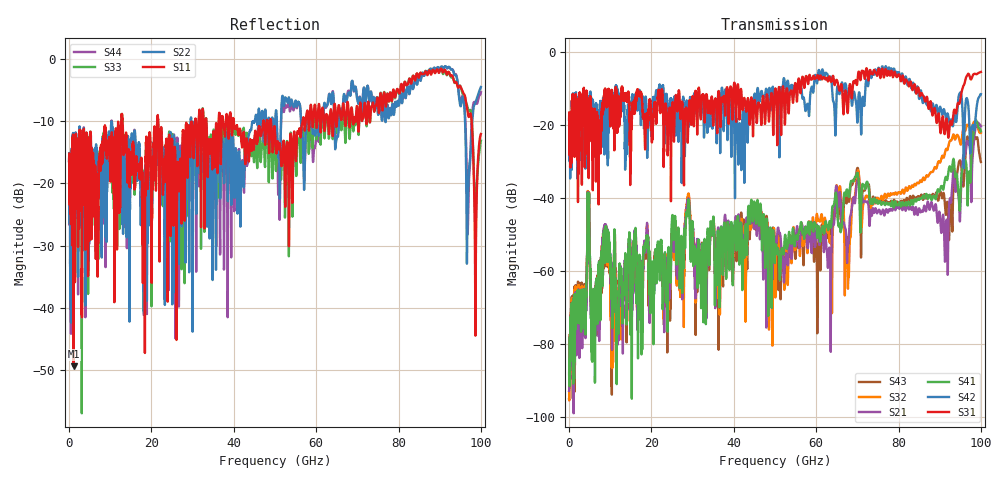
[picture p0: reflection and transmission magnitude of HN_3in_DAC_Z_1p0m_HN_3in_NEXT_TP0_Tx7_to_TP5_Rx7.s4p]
# GHz S RI R 45
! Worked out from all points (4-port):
!   4000 points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, 25 MHz to 100 GHz, reference 45 ohm
!   strongest paths, dB at 25 MHz, 25.02 GHz, 50.02 GHz, 75.03 GHz, 100 GHz:
!     S31: -18.6, -14.9, -10.3, -5.2, -5.5
!     S42: -18.6, -16.6, -12.4, -4.6, -11.5
!     S41: -88.3, -45.2, -55.9, -41.6, -21.7
!     S21: -92.8, -49.6, -53.3, -43.6, -20.4
!     S32: -95.1, -50.6, -58.0, -40.0, -22.2
!     S43: -95.0, -46.6, -57.9, -40.4, -30.1
!   lowest |S11| = -49.4 dB at 1.125 GHz (marker M1), VSWR 1.01, Z = 44.8 + j0.19 ohm
!   |S11| at or under -10 dB: start of sweep to 12.67 GHz; 12.99 GHz to 21.42 GHz (8.433 GHz wide, 49 % of centre); 21.66 GHz to 30.61 GHz (8.947 GHz wide, 34.2 % of centre)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
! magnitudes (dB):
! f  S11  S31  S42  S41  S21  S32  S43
! 25 MHz  -16.5  -18.6  -18.6  -88.3  -92.8  -95.1  -95.0
! 1.125 GHz  -49.4  -24.2  -21.7  -85.1  -99.0  -82.9  -81.7
! 28.85 GHz  -17.2  -24.1  -15.4  -43.3  -40.8  -39.7  -41.2
! 51.17 GHz  -13.6  -10.9  -18.7  -62.4  -49.7  -49.8  -61.1
! 67.45 GHz  -7.7  -13.7  -11.1  -37.6  -56.1  -50.8  -41.3
! 91.58 GHz  -2.3  -18.6  -18.2  -34.2  -46.7  -26.5  -44.1
! 100 GHz  -12.1  -5.5  -11.5  -21.7  -20.4  -22.2  -30.1
